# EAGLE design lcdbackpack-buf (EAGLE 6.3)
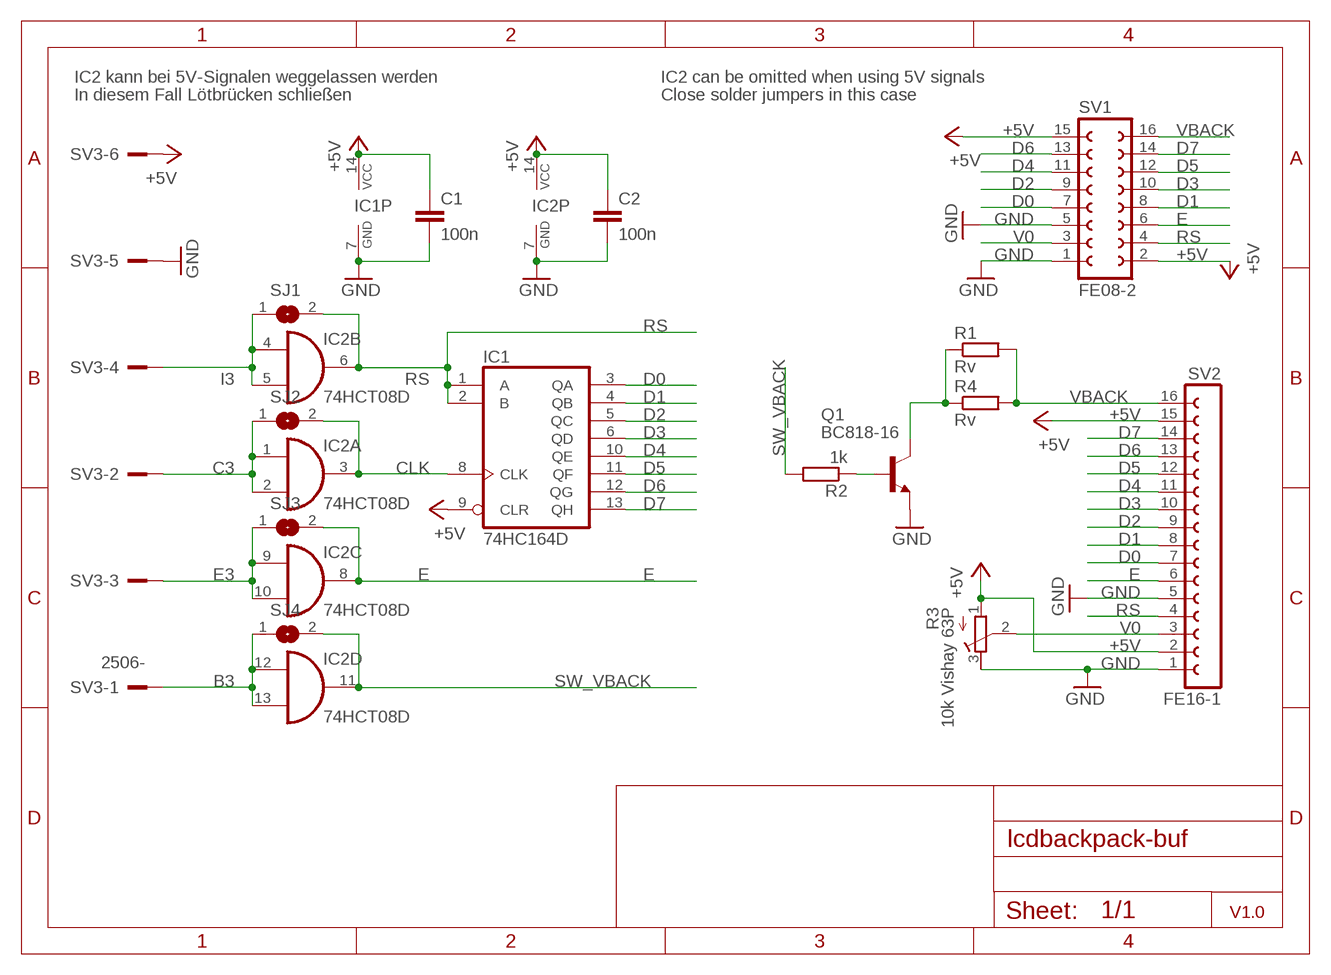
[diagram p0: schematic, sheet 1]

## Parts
C1  100n  C-EUC0603  [C0603]
C2  100n  C-EUC0603  [C0603]
IC1  74HC164D  [SO14]
IC2  74HCT08D  [SO14]
Q1  BC818-16  BC818-16SMD  [SOT23-BEC]
R1  Rv  R-EU_R0805  [R0805]
R2  1k  R-EU_R0603  [R0603]
R3  10k Vishay 63P  R-TRIMM3339P  [RTRIM3339P]
R4  Rv  R-EU_R0805  [R0805]
SJ1  SJ  [SJ]
SJ2  SJ  [SJ]
SJ3  SJ  [SJ]
SJ4  SJ  [SJ]
SV1  FE08-2  [FE08-2]
SV2  FE16-1  [FE16]
SV3  2506-  [PAK100/2500-06]

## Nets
+5V: C1.1 C2.1 IC1.9(CLR) IC1.14(VCC) IC2.14(P:VCC) R3.1(A) SV1.2 SV1.15 SV2.2 SV2.15 SV3.6
B3: IC2.12(D:I0) IC2.13(D:I1) SJ4.1 SV3.1
C3: IC2.1(A:I0) IC2.2(A:I1) SJ2.1 SV3.2
CLK: IC1.8(CLK) IC2.3(A:O) SJ2.2
D0: IC1.3(QA) SV1.7 SV2.7
D1: IC1.4(QB) SV1.8 SV2.8
D2: IC1.5(QC) SV1.9 SV2.9
D3: IC1.6(QD) SV1.10 SV2.10
D4: IC1.10(QE) SV1.11 SV2.11
D5: IC1.11(QF) SV1.12 SV2.12
D6: IC1.12(QG) SV1.13 SV2.13
D7: IC1.13(QH) SV1.14 SV2.14
E: IC2.8(C:O) SJ3.2 SV1.6 SV2.6
E3: IC2.9(C:I0) IC2.10(C:I1) SJ3.1 SV3.3
GND: C1.2 C2.2 IC1.7(GND) IC2.7(P:GND) Q1.E R3.3(E) SV1.1 SV1.5 SV2.1 SV2.5 SV3.5
I3: IC2.4(B:I0) IC2.5(B:I1) SJ1.1 SV3.4
RS: IC1.1(A) IC1.2(B) IC2.6(B:O) SJ1.2 SV1.4 SV2.4
SW_VBACK: IC2.11(D:O) R2.2 SJ4.2
SW_VBACK1: Q1.B R2.1
V0: R3.2(S) SV1.3 SV2.3
VBACK: R1.2 R4.2 SV1.16 SV2.16
VBACK_R: Q1.C R1.1 R4.1

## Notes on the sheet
- IC2 kann bei 5V-Signalen weggelassen werden | IC2 can be omitted when using 5V signals
- In diesem Fall Lötbrücken schließen | Close solder jumpers in this case
- V1.0

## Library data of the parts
C1 C2 = rcl:C-EU: CAPACITOR, European symbol
IC1 = 74xx-eu:74*164: 8-bit parallel out SHIFT REGISTER
IC2 = 74xx-eu:74*08: Quad 2-input AND gate
Q1 = transistor-npn:BC818*: NPN Transistor
R1 R2 R4 = rcl:R-EU_: RESISTOR, European symbol
R3 = rcl:R-TRIMM: Trimm resistor
SJ1-SJ4 = fchk:SJ: SMD solder JUMPER
SV1 = con-lsta2:FE08-2: FEMALE HEADER
SV2 = con-lsta2:FE16-1: FEMALE HEADER
SV3 = con-3m:2506-: 3M (TM) Pak 100 4-Wall Header Source: 3M

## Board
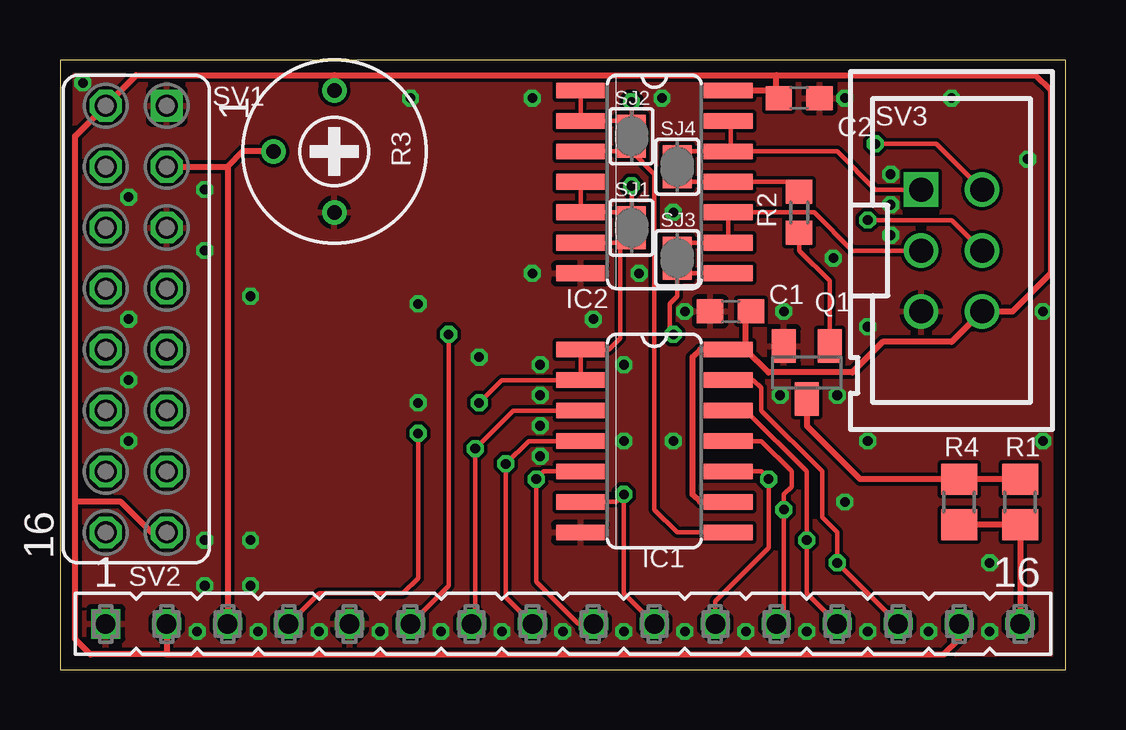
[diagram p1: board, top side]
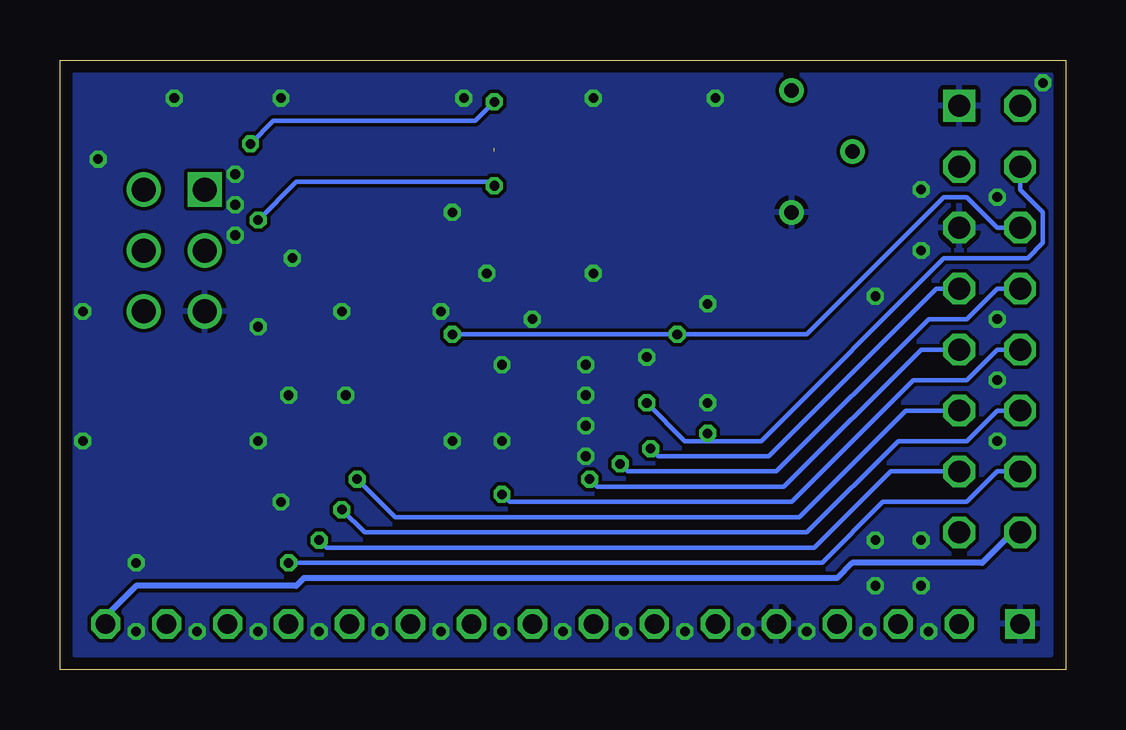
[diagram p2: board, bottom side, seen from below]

Size 41.91 x 25.4 mm. Coordinates in mm from the lower left corner, seen from the top.
Outline: 0,0 41.91,0 41.91,25.4 0,25.4 0,0
Copper layers (1+2*15+16): Top 0.035mm / dielectric 0.36mm / Route2 0.035mm / dielectric 0.71mm / Route15 0.035mm / dielectric 0.36mm / Bottom 0.035mm
Design rules "default": minimum track width 6mil, minimum drill 0.3mm, track to track 6mil, track to pad 6mil, pad to pad 6mil, via to via 6mil, smd to smd 6mil, copper to edge 20mil, drill to drill 10mil, minimum pad ring 8mil, minimum via ring 6mil, stop-mask expansion 3mil, vias tented up to drill 0mil, thermal gap 8mil

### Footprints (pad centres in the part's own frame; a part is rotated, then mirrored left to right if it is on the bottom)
C0603 = smd 1.1 x 1: 1 -0.85,0; 2 0.85,0
SO14 = smd 0.66 x 2.032: 1 -3.81,-3.073; 2 -2.54,-3.073; 3 -1.27,-3.073; 4 0,-3.073; 5 1.27,-3.073; 6 2.54,-3.073; 7 3.81,-3.073; 8 3.81,3.073; 9 2.54,3.073; 10 1.27,3.073; 11 0,3.073; 12 -1.27,3.073; 13 -2.54,3.073; 14 -3.81,3.073
SOT23-BEC = smd 1 x 1.4: B -0.95,-1.1; C 0,1.1; E 0.95,-1.1
R0805 = smd 1.3 x 1.5: 1 -0.95,0; 2 0.95,0
R0603 = smd 1 x 1.1: 1 -0.85,0; 2 0.85,0
RTRIM3339P = drill 0.61: 1 -2.54,0; 2 0,-2.54; 3 2.54,0
SJ = smd 0.8 x 1.2: 1 -0.5,0; 2 0.5,0
FE08-2 = drill 0.914 square: 1 -8.89,1.27 | drill 0.914 octagon: 2 -8.89,-1.27; 3 -6.35,1.27; 4 -6.35,-1.27; 5 -3.81,1.27; 6 -3.81,-1.27; 7 -1.27,1.27; 8 -1.27,-1.27; 9 1.27,1.27; 10 1.27,-1.27; 11 3.81,1.27; 12 3.81,-1.27; 13 6.35,1.27; 14 6.35,-1.27; 15 8.89,1.27; 16 8.89,-1.27
FE16 = drill 0.813 square: 1 -19.05,0 | drill 0.813 octagon: 2 -16.51,0; 3 -13.97,0; 4 -11.43,0; 5 -8.89,0; 6 -6.35,0; 7 -3.81,0; 8 -1.27,0; 9 1.27,0; 10 3.81,0; 11 6.35,0; 12 8.89,0; 13 11.43,0; 14 13.97,0; 15 16.51,0; 16 19.05,0
PAK100/2500-06 = drill 1 pad 1.422 square: 1 -2.54,-1.27 | drill 1 pad 1.422: 2 -2.54,1.27; 3 0,-1.27; 4 0,1.27; 5 2.54,-1.27; 6 2.54,1.27

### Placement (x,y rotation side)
C1  27.94,14.92 180 top
C2  30.8,23.81 0 top
IC1  24.77,9.53 270 top
IC2  24.77,20.32 270 top
Q1  31.11,12.38 180 top
R1  40.01,6.99 270 top
R2  30.8,19.05 90 top
R3  11.43,21.59 270 top
R4  37.47,6.99 270 top
SJ1  23.81,18.41 270 top
SJ2  23.81,22.23 270 top
SJ3  25.72,17.14 270 top
SJ4  25.72,20.95 270 top
SV1  3.17,14.61 270 top
SV2  20.95,1.91 0 top
SV3  37.15,17.46 270 top

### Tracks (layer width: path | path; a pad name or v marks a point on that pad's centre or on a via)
+5V
  Top 0.254: IC2.14 29.95,24.13 C2.1 29.84,23.91 29.84,24.77 | 28.57,13.34 IC1.14 26.67,13.34 26.35,13.02 26.35,7.3 26.67,6.99 IC1.9 | 28.57,13.34 28.57,14.92 C1.1 | 11.43,24.77 3.17,24.77 SV1.2 0.64,22.23 0.64,6.99 | 11.43,24.77 29.84,24.77 | 29.84,24.77 40.64,24.77 41.27,24.13 41.27,16.51 39.69,14.92 SV3.6 37.15,13.65 34.29,13.65 33.02,12.38 29.53,12.38 28.57,13.34 | SV2.2 4.45,0.64 | 4.45,0.64 1.27,0.64 0.64,1.27 0.64,6.99 | SV1.15 3.81,5.71 2.54,6.99 0.64,6.99 | 4.45,0.64 36.83,0.64 37.47,1.27 SV2.15 | R3.1 11.43,24.77
B3
  Top 0.178: IC2.13 27.94,22.76 27.94,21.59 | SV3.1 33.97,20 32.38,21.59 27.94,21.59 | 27.94,21.59 IC2.12 25.85,21.59 SJ4.1
C3  (via drill 0.4)
  Top 0.178: IC2.1 IC2.2 23.5,22.86 23.63,22.73 SJ2.1 v23.81,23.65 | SV3.2 36.51,21.91 v33.97,21.91
  Bottom 0.178: v33.97,21.91 33.02,22.86 24.61,22.86 v23.81,23.65
CLK  (1 unrouted)
  Top 0.178: IC2.3 23.81,21.59 24.77,20.64 24.77,6.67 25.72,5.71 IC1.8
D0  (via drill 0.4)
  Top 0.178: IC1.3 18.89,10.79 v17.3,9.21 17.3,2.06 SV2.7
  Bottom 0.178: SV1.7 5.4,15.88 12.38,8.89 16.99,8.89 v17.3,9.21
D1  (via drill 0.4)
  Top 0.178: IC1.4 19.53,9.53 v18.57,8.57 18.57,3.02 SV2.8
  Bottom 0.178: SV1.8 2.86,15.88 4.13,14.61 5.71,14.61 12.06,8.26 18.26,8.26 v18.57,8.57
D2  (via drill 0.4)
  Top 0.178: SV2.9 21.59,1.91 19.84,3.65 v19.84,7.94 20.16,8.26 IC1.5
  Bottom 0.178: SV1.9 6.03,13.34 11.75,7.62 19.53,7.62 v19.84,7.94
D3  (via drill 0.4)
  Top 0.178: IC1.6 23.18,6.99 v23.5,7.3 23.5,3.17 SV2.10
  Bottom 0.178: SV1.10 2.86,13.34 4.13,12.06 6.35,12.06 11.43,6.99 23.18,6.99 v23.5,7.3
D4  (via drill 0.4)
  Top 0.178: SV2.11 27.3,2.86 29.53,5.08 v29.53,7.94 29.21,8.26 IC1.10
  Bottom 0.178: SV1.11 6.67,10.79 11.11,6.35 27.94,6.35 v29.53,7.94
D5  (via drill 0.4)
  Top 0.178: IC1.11 29.21,9.53 30.48,8.26 30.48,7.62 30.16,7.3 v30.16,6.67 30.16,2.22 SV2.12
  Bottom 0.178: SV1.12 2.86,10.79 4.13,9.53 6.99,9.53 10.79,5.71 29.21,5.71 v30.16,6.67
D6  (via drill 0.4)
  Top 0.178: IC1.12 28.57,10.79 31.11,8.26 v31.11,5.4 31.11,3.17 SV2.13
  Bottom 0.178: SV1.13 7.3,8.26 10.48,5.08 30.8,5.08 v31.11,5.4
D7  (via drill 0.4)
  Top 0.178: IC1.13 28.89,12.06 29.21,11.75 29.21,10.79 31.75,8.26 31.75,6.35 32.38,5.71 v32.38,4.45 SV2.14
  Bottom 0.178: SV1.14 2.86,8.26 4.13,6.99 7.62,6.99 10.16,4.45 v32.38,4.45
E  (via drill 0.4)
  Top 0.178: SV2.6 16.19,3.49 v16.19,13.97 | IC2.8 25.85,16.51 SJ3.2 25.72,15.56 25.4,15.24 25.4,14.13 v25.56,13.97
  Bottom 0.178: SV1.6 2.86,18.41 4.13,19.68 5.08,19.68 10.79,13.97 v16.19,13.97 v25.56,13.97
E3
  Top 0.178: SV3.3 33.02,17.46 31.43,19.05 IC2.10 IC2.9 25.85,17.78 SJ3.1
GND  (via drill 0.4)
  other vias: 26.04,14.92 14.61,23.81 20,11.43 23.5,9.53 34.61,20.64 20,8.89 40.32,21.27 34.61,19.37 34.61,18.1 24.13,16.51 20.95,1.59 23.5,1.59 26.04,1.59 28.57,1.59 31.11,1.59 33.66,1.59 36.2,1.59 18.41,1.59 15.88,1.59 13.34,1.59 10.79,1.59 8.26,1.59 7.94,15.56 2.86,12.06 2.86,9.53 2.86,14.61 2.86,19.68 0.95,24.45 7.94,5.4 40.96,14.92 23.5,12.7 19.68,16.51 32.7,23.81 37.15,23.81 5.71,1.59 6.03,17.46 7.94,3.49 25.56,9.53 32.38,11.43 30.16,14.92 25.08,23.81 20,12.7 6.03,20 19.68,23.81 40.96,9.53 22.23,14.61 20,10.16 14.92,15.24 14.92,11.11 17.46,13.02 6.03,3.49 6.03,5.4 38.73,1.59 32.7,6.99 38.73,4.45 25.56,19.05 32.23,17.14 33.66,14.29 30,11.43 33.66,9.53
  pour Bottom (rank 6): 41.27,0.64 0.64,0.64 0.64,24.77 41.27,24.77
  pour Top (rank 6): 0.64,24.77 41.27,24.77 41.27,0.64 0.64,0.64
  pour Top (no thermals): 8.26,17.78 12.7,17.78 12.7,3.81 8.26,3.81
  pour Bottom (no thermals): 34.92,23.81 39.37,23.81 39.37,20.95 34.92,20.95
  pour Bottom (no thermals): 33.34,17.78 34.92,17.78 34.92,16.19 33.34,16.19
  pour Bottom (no thermals): 34.92,13.65 39.37,13.65 39.37,9.84 34.92,9.84
  pour Bottom (no thermals): 39.05,19.05 41.27,19.05 41.27,16.83 39.05,16.83
I3  (via drill 0.4)
  Top 0.178: IC2.4 IC2.5 23.68,19.05 SJ1.1 v23.81,20.16 | SV3.4 37.15,18.73 v33.66,18.73
  Bottom 0.178: v33.66,18.73 32.07,20.32 23.97,20.32 v23.81,20.16
RS  (via drill 0.4)
  Top 0.178: v17.46,11.11 18.41,12.06 IC1.2 IC1.1 22.86,13.34 23.34,13.81 23.34,17.78 | IC2.6 23.34,17.78 | SV2.4 10.79,3.17 14.29,3.17 14.92,3.81 v14.92,9.84 | SJ1.2 23.68,17.78 23.34,17.78
  Bottom 0.178: SV1.4 1.91,20 0.95,19.05 0.95,17.78 1.59,17.14 5.08,17.14 12.7,9.53 14.92,9.53 | 14.92,9.53 15.88,9.53 v17.46,11.11 | v14.92,9.84 14.92,9.53
SW_VBACK
  Top 0.178: R2.2 30.8,20.32 IC2.11 25.85,20.32 SJ4.2
SW_VBACK1
  Top 0.178: R2.1 30.8,17.46 32.07,16.19 Q1.B
V0
  Top 0.254: R3.2 7.62,21.59 6.99,20.95 | 6.99,20.95 SV2.3 | SV1.3 6.99,20.95
VBACK
  Top 0.254: SV2.16 R1.2 R4.2
  Bottom 0.254: SV1.16 2.22,5.71 3.49,4.45 8.89,4.45 9.53,3.81 31.75,3.81 32.07,3.49 38.73,3.49 40.01,2.22 SV2.16
VBACK_R
  Top 0.254: Q1.C 31.11,10.16 33.34,7.93 R4.1 R1.1

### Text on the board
tRestrict: VER 1.0 | LCDBACKPACK
bRestrict: BL | CK | E | SI | GND | +5V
